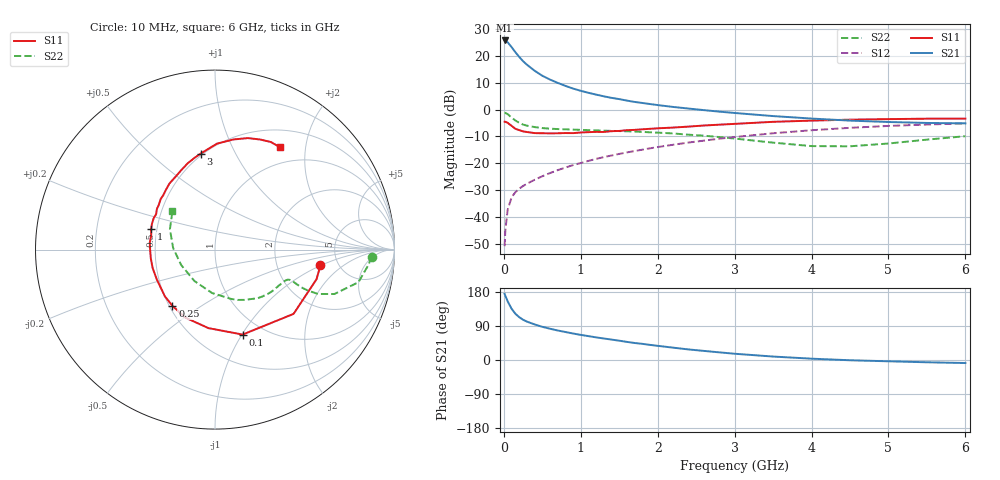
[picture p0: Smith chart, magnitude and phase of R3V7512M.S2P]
! SIEMENS Small Signal Semiconductors
! BFR181
! Si NPN RF Bipolar Junction Transistor in SOT23
! VCE = 0.75 V  IC = 12 mA
! Common Emitter S-Parameters:  May  1996
# GHz  S  MA  R  50
!  f  S11  S21  S12  S22
! GHz  MAG  ANG  MAG  ANG  MAG  ANG  MAG  ANG
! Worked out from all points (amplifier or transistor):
!   36 points, 10 MHz to 6 GHz, reference 50 ohm
!   highest |S21| = 25.6 dB at 10 MHz (marker M1)
!   |S21| within 3 dB of that: start of sweep to 114.4 MHz
!   unconditionally stable (mu >= 1): start of sweep to 15.48 MHz; 238.9 MHz to end of sweep
!   at 250 MHz: K = 1.03, MAG = 22.1 dB, |S12| = -28.4 dB
!   at 1.4 GHz: K = 1.50, MAG = 6.5 dB, |S12| = -17.1 dB
!   at 6 GHz: K = 1.16, MAG = -2.4 dB, |S12| = -5.2 dB
!   S11 on the Smith chart (normalised r, x): 10 MHz: 3.64, -0.99; 100 MHz: 0.80, -1.01; 250 MHz: 0.52, -0.38; 1 GHz: 0.46, +0.12; 3 GHz: 0.49, +0.74; 6 GHz: 0.74, +1.55
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0.01  0.5942 -8.5  19.14 174.6  0.0029 81.1  0.8731 -2.6
0.02  0.5892 -16.3  18.85 169.2  0.0058 81.6  0.8604 -5.5
0.05  0.5655 -39.3  17.66 154.7  0.0138 72.2  0.8197 -12.8
0.1  0.4977 -72.0  14.45 135.5  0.0233 63.2  0.7099 -20.4
0.15  0.439 -94.8  11.58 122.0  0.0292 57.4  0.625 -23.3
0.2  0.4135 -113.7  9.474 113.0  0.0339 56.9  0.5651 -23.8
0.25  0.3928 -127.1  7.885 106.2  0.038 56.7  0.5253 -23.6
0.3  0.3818 -137.0  6.787 101.3  0.0418 58.4  0.501 -23.1
0.4  0.3645 -152.9  5.249 93.9  0.0496 60.0  0.4716 -22.3
0.5  0.3622 -163.9  4.234 87.5  0.0576 62.3  0.4523 -22.0
0.6  0.361 -172.5  3.595 82.5  0.066 63.8  0.4402 -22.3
0.7  0.3617 179.3  3.124 77.9  0.0748 65.3  0.4334 -23.0
0.9  0.3641 167.5  2.447 69.9  0.0929 66.1  0.4237 -24.8
1  0.3741 162.1  2.223 66.3  0.1015 66.7  0.4183 -26.2
1.1  0.3798 157.5  2.04 63.0  0.1112 66.6  0.4139 -27.7
1.6  0.413 137.2  1.463 47.8  0.1597 64.9  0.3939 -36.1
2.2  0.4617 118.4  1.116 32.6  0.2215 60.5  0.3593 -49.1
3  0.541 98.5  0.862 16.5  0.3078 51.9  0.2888 -72.0
3.5  0.5905 88.9  0.755 9.1  0.362 45.5  0.2424 -93.9
4.5  0.6476 73.6  0.622 -0.7  0.4572 30.9  0.2074 -155.9
5.5  0.6753 62.6  0.563 -6.0  0.5264 16.7  0.2758 155.6
6  0.6757 57.8  0.553 -8.0  0.5514 9.5  0.3193 138.0
